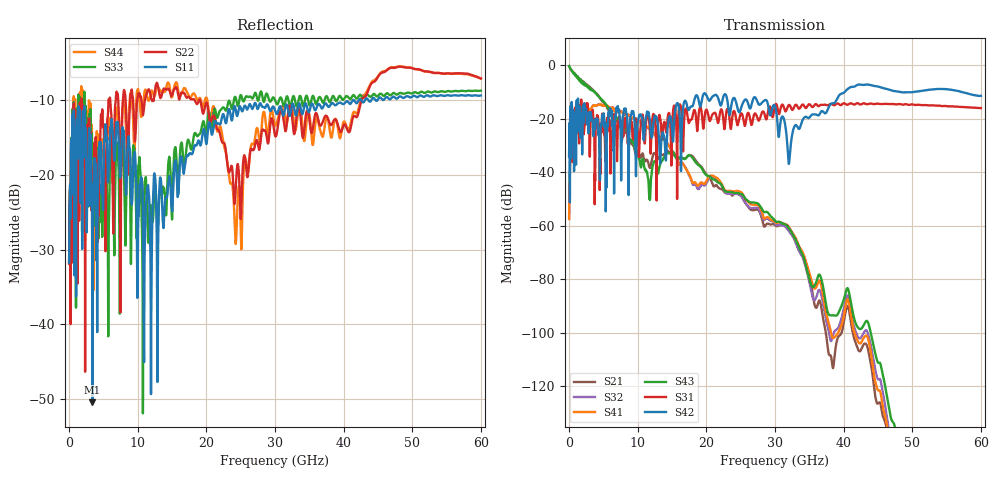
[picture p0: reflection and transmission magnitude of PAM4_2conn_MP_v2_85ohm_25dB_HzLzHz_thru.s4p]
! Info: Touchstone file created by Circ.  Input file=FAB50GbE_2conn_Midplane_Examax_Topo2_v2_85ohm_25dB_HzLzHz.circ
# Hz S RI R 50
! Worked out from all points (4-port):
!   6000 points, 10 MHz to 60 GHz, reference 50 ohm
!   strongest paths, dB at 10 MHz, 15.01 GHz, 30.01 GHz, 45.01 GHz, 60 GHz:
!     S42: -34.0, -24.0, -15.3, -7.9, -11.4
!     S31: -34.1, -23.4, -14.9, -14.3, -16.0
!     S43: -0.3, -32.0, -58.1, -111.2, -179.4
!     S41: -57.5, -32.5, -58.6, -121.6, -179.3
!     S32: -57.5, -32.7, -59.2, -117.5, -170.1
!     S21: -0.3, -32.2, -59.8, -126.6, -166.7
!   lowest |S11| = -50.5 dB at 3.4 GHz (marker M1), VSWR 1.01, Z = 49.8 + j0.178 ohm
!   |S11| at or under -10 dB: start of sweep to 41.32 GHz; 41.55 GHz to 42.2 GHz (645.9 MHz wide, 1.54 % of centre); 42.59 GHz to 43.11 GHz (522.1 MHz wide, 1.22 % of centre)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
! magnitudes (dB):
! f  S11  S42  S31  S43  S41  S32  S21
! 10 MHz  -31.7  -34.0  -34.1  -0.3  -57.5  -57.5  -0.3
! 810 MHz  -20.2  -27.1  -20.2  -3.1  -18.5  -18.3  -3.0
! 3.4 GHz  -50.5  -20.3  -17.0  -9.2  -15.4  -15.4  -8.9
! 11.68 GHz  -23.2  -19.5  -21.5  -49.8  -23.5  -23.7  -37.9
! 17.69 GHz  -17.1  -15.5  -20.3  -33.8  -41.8  -42.2  -33.6
! 35.24 GHz  -10.7  -18.8  -15.1  -81.9  -79.8  -84.0  -81.4
! 60 GHz  -9.3  -11.4  -16.0  -179.4  -179.3  -170.1  -166.7
